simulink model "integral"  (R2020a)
settings: Solver=ode45  StartTime=-1  StopTime=6.0  RelTol=1e-14  EnableMultiTasking=on

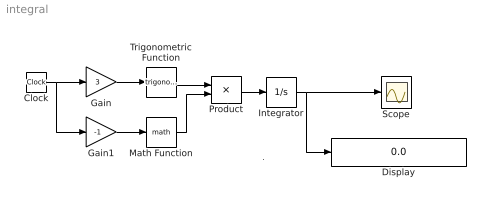
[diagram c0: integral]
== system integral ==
  note: .
  Clock : Clock
  Display : Display
  Gain : Gain  Gain=3  SaturateOnIntegerOverflow=on
  Gain1 : Gain  Gain=-1  SaturateOnIntegerOverflow=on
  Integrator : Integrator
  Math Function : Math  SignedPower=on
  Product : Product  InputSameDT=on  SaturateOnIntegerOverflow=on
  Scope : Scope
  Trigonometric Function : Trigonometry
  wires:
  Gain/1 -> Trigonometric Function/1
  Clock/1 -> Gain/1, Gain1/1
  Trigonometric Function/1 -> Product/1
  Gain1/1 -> Math Function/1
  Math Function/1 -> Product/2
  Product/1 -> Integrator/1
  Integrator/1 -> Scope/1, Display/1
